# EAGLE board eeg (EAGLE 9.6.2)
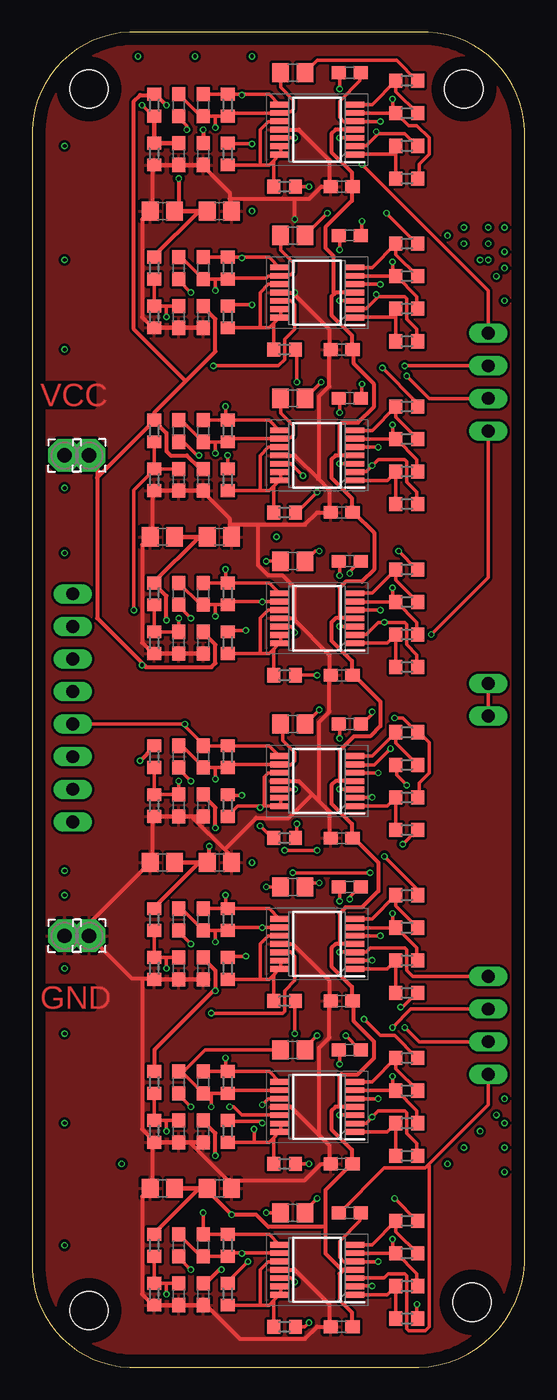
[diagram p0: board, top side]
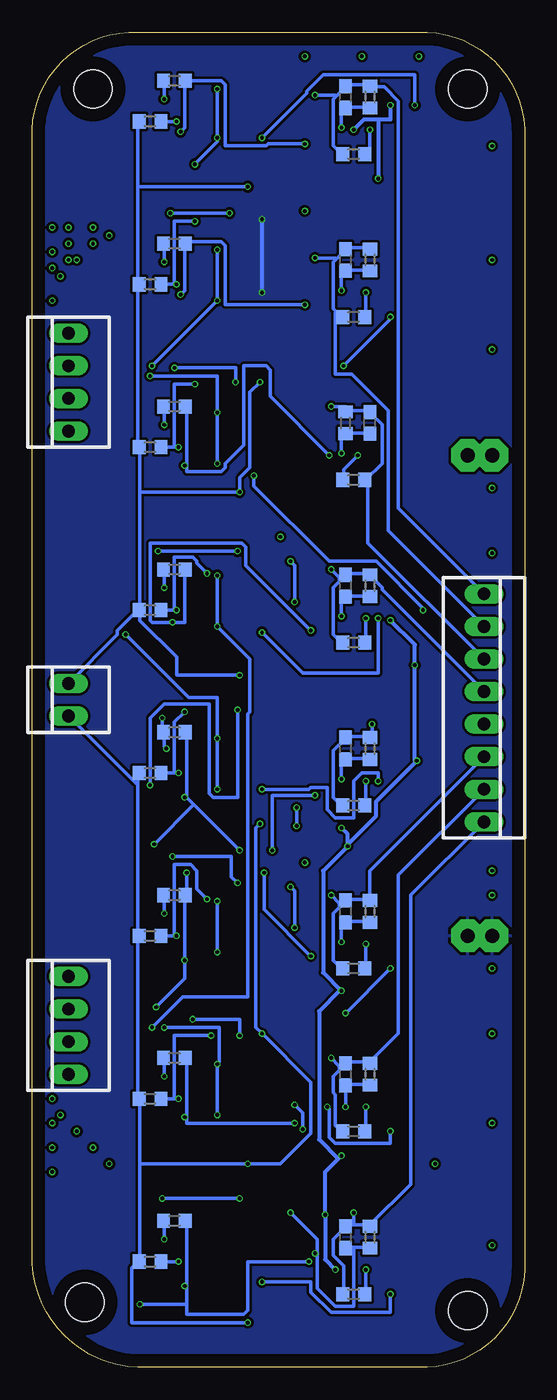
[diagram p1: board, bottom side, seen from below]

Size 38.4 x 104.13 mm. Coordinates in mm from the lower left corner, seen from the top.
Outline: 0,95.88 0,8.26 arc90 7.62,0 30.15,0 arc90 38.4,8.89 38.4,96.51 arc90 30.15,104.13 7.62,104.13 arc90 0,95.88
Copper layers (1*16): Top 0.035mm / dielectric 1.5mm / Bottom 0.035mm
Design rules "default *": minimum track width 10mil, minimum drill 0.3mm, track to track 6mil, track to pad 6mil, pad to pad 6mil, via to via 6mil, smd to smd 6mil, copper to edge 40mil, drill to drill 6mil, minimum pad ring 10mil, minimum via ring 2mil, stop-mask expansion 4mil, vias tented up to drill 0mil, thermal gap 10mil
Net classes: 0 default: width 0.254 mm, drill 0.3 mm, clearance 0.205 mm; 1 VCC: width 0.305 mm, drill 0.3 mm, clearance 0.205 mm; 2 GND: width 0.305 mm, drill 0.3 mm, clearance 0.205 mm
Holes 3 mm at 4.45,4.45 34.29,5.08 33.65,99.7 4.45,99.7

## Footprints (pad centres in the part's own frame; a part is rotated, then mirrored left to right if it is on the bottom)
22-23-2081 = drill 1 long: 1 -8.89,0; 2 -6.35,0; 3 -3.81,0; 4 -1.27,0; 5 1.27,0; 6 3.81,0; 7 6.35,0; 8 8.89,0
R0603 = smd 1 x 1.1: 1 -0.85,0; 2 0.85,0
C0603 = smd 1.1 x 1: 1 -0.85,0; 2 0.85,0
C0805 = smd 1.3 x 1.5: 1 -0.95,0; 2 0.95,0
22-23-2041 = drill 1 long: 1 -3.81,0; 2 -1.27,0; 3 1.27,0; 4 3.81,0
SOP65P640X120-14N = smd 1.475 x 0.45: 1 -2.938,1.95; 2 -2.938,1.3; 3 -2.938,0.65; 4 -2.938,0; 5 -2.938,-0.65; 6 -2.938,-1.3; 7 -2.938,-1.95; 8 2.938,-1.95; 9 2.938,-1.3; 10 2.938,-0.65; 11 2.938,0; 12 2.938,0.65; 13 2.938,1.3; 14 2.938,1.95
2,54/1,1 = drill 1.118 pad 2.54 octagon: 1 0,0
22-23-2021 = drill 1 long: 1 -1.27,0; 2 1.27,0

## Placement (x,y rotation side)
ANALOGOUT  22-23-2081  [22-23-2081]  3.18,51.44 270 bottom
BANDPASS  [R0603]  13.34,94.61 0 bottom
BANDPASS1  [R0603]  13.34,81.92 0 bottom
BANDPASS2  [R0603]  13.34,69.22 180 bottom
BANDPASS3  [R0603]  13.34,56.52 0 bottom
BANDPASS4  [R0603]  13.34,43.82 0 bottom
BANDPASS5  [R0603]  13.34,31.12 0 bottom
BANDPASS6  [R0603]  13.34,18.41 0 bottom
BANDPASS7  [R0603]  13.34,5.71 0 bottom
C1  [C0603]  24.77,100.97 0 top
C2  [C0603]  24.13,92.08 180 top
C3  [C0805]  20.32,100.97 0 top
C4  [C0603]  13.34,98.42 90 top
C5  [C0603]  13.34,94.61 270 top
C6  [C0603]  11.43,98.42 270 top
C7  [C0603]  11.43,94.61 270 top
C8  [C0805]  20.32,88.27 0 top
C9  [C0603]  24.77,88.27 0 top
C10  [C0603]  24.13,79.38 180 top
C11  [C0603]  13.34,81.92 270 top
C12  [C0603]  11.43,85.73 270 top
C13  [C0603]  13.34,85.73 90 top
C14  [C0603]  11.43,81.92 270 top
C15  [C0805]  20.32,75.56 0 top
C16  [C0603]  24.77,75.56 0 top
C17  [C0603]  24.13,66.67 180 top
C18  [C0603]  13.34,69.22 270 top
C19  [C0603]  11.43,73.03 270 top
C20  [C0603]  13.34,73.03 90 top
C21  [C0603]  11.43,69.22 270 top
C22  [C0805]  20.32,62.86 0 top
C23  [C0603]  24.77,62.86 0 top
C24  [C0603]  24.13,53.98 180 top
C25  [C0603]  13.34,56.52 270 top
C26  [C0603]  11.43,60.33 270 top
C27  [C0603]  13.34,60.33 90 top
C28  [C0603]  11.43,56.52 270 top
C29  [C0805]  20.32,50.16 0 top
C30  [C0603]  24.77,50.16 0 top
C31  [C0603]  24.13,41.27 180 top
C32  [C0603]  13.34,43.82 270 top
C33  [C0603]  11.43,47.62 270 top
C34  [C0603]  13.34,47.62 90 top
C35  [C0603]  11.43,43.82 270 top
C36  [C0805]  20.32,37.47 0 top
C37  [C0603]  24.77,37.47 0 top
C38  [C0603]  24.13,28.58 180 top
C39  [C0603]  13.34,31.12 270 top
C40  [C0603]  11.43,34.93 270 top
C41  [C0603]  13.34,34.93 90 top
C42  [C0603]  11.43,31.12 270 top
C43  [C0805]  20.32,24.77 0 top
C44  [C0603]  24.77,24.77 0 top
C45  [C0603]  24.13,15.87 180 top
C46  [C0603]  13.34,18.41 270 top
C47  [C0603]  11.43,22.23 270 top
C48  [C0603]  13.34,22.23 90 top
C49  [C0603]  11.43,18.41 270 top
C50  [C0805]  20.32,12.06 0 top
C51  [C0603]  24.77,12.06 0 top
C52  [C0603]  13.34,5.71 270 top
C53  [C0603]  24.13,3.18 180 top
C54  [C0603]  11.43,9.53 270 top
C55  [C0603]  13.34,9.53 90 top
C56  [C0603]  11.43,5.71 270 top
C59  [C0805]  10.16,90.17 180 top
C60  [C0805]  14.61,90.17 180 top
C61  [C0805]  10.16,64.77 180 top
C62  [C0805]  14.61,64.77 180 top
C63  [C0805]  10.16,39.37 180 top
C64  [C0805]  14.61,39.37 180 top
C65  [C0805]  10.16,13.97 180 top
C66  [C0805]  14.61,13.97 180 top
E$1  [22-23-2041]  35.56,76.84 90 bottom
E$2  [22-23-2041]  35.56,26.67 90 bottom
FILTERC  [C0603]  13.97,99.06 90 bottom
FILTERC1  [C0603]  13.97,86.36 90 bottom
FILTERC2  [C0603]  12.07,73.66 90 bottom
FILTERC3  [C0603]  13.97,60.96 90 bottom
FILTERC4  [C0603]  13.97,48.26 90 bottom
FILTERC5  [C0603]  13.97,35.56 90 bottom
FILTERC6  [C0603]  13.97,22.86 90 bottom
FILTERC7  [C0603]  13.97,10.16 90 bottom
FILTERR  [R0603]  12.07,99.06 270 bottom
FILTERR1  [R0603]  12.07,86.36 270 bottom
FILTERR2  [R0603]  13.97,73.66 270 bottom
FILTERR3  [R0603]  12.07,60.96 270 bottom
FILTERR4  [R0603]  12.07,48.26 270 bottom
FILTERR5  [R0603]  12.07,35.56 270 bottom
FILTERR6  [R0603]  12.07,22.86 270 bottom
FILTERR7  [R0603]  12.07,10.16 270 bottom
GAIN  [R0603]  27.3,100.33 180 bottom
GAIN1  [R0603]  27.3,87.63 180 bottom
GAIN2  [R0603]  27.3,74.93 180 bottom
GAIN3  [R0603]  27.3,62.23 180 bottom
GAIN4  [R0603]  27.3,49.53 180 bottom
GAIN5  [R0603]  27.3,36.83 180 bottom
GAIN6  [R0603]  27.3,24.13 180 bottom
GAIN7  [R0603]  27.3,11.43 180 bottom
IC1  ADTL084ARUZ  [SOP65P640X120-14N]  22.23,96.52 180 top
IC2  ADTL084ARUZ  [SOP65P640X120-14N]  22.23,83.82 180 top
IC3  ADTL084ARUZ  [SOP65P640X120-14N]  22.23,71.12 180 top
IC4  ADTL084ARUZ  [SOP65P640X120-14N]  22.23,58.42 180 top
IC5  ADTL084ARUZ  [SOP65P640X120-14N]  22.23,45.72 180 top
IC6  ADTL084ARUZ  [SOP65P640X120-14N]  22.23,33.02 180 top
IC7  ADTL084ARUZ  [SOP65P640X120-14N]  22.23,20.32 180 top
IC8  ADTL084ARUZ  [SOP65P640X120-14N]  22.23,7.62 180 top
PAD1  [2,54/1,1]  2.54,33.66 90 top
PAD2  [2,54/1,1]  4.45,33.66 90 top
PAD3  [2,54/1,1]  2.54,71.12 90 top
PAD4  [2,54/1,1]  4.45,71.12 90 top
R1  [R0603]  29.21,100.33 180 top
R2  [R0603]  29.21,97.79 0 top
R3  [R0603]  29.21,87.63 180 top
R4  [R0603]  29.21,85.09 0 top
R5  [R0603]  29.21,95.25 180 top
R6  [R0603]  29.21,92.71 180 top
R7  [R0603]  19.68,92.08 180 top
R8  [R0603]  15.24,98.42 270 top
R9  [R0603]  15.24,94.61 270 top
R10  [R0603]  9.53,98.42 270 top
R11  [R0603]  9.53,94.61 270 top
R12  [R0603]  29.21,82.55 180 top
R13  [R0603]  29.21,80.01 180 top
R14  [R0603]  15.24,81.92 270 top
R15  [R0603]  15.24,85.73 270 top
R16  [R0603]  9.53,85.73 270 top
R17  [R0603]  9.53,81.92 270 top
R18  [R0603]  19.68,79.38 180 top
R19  [R0603]  29.21,74.93 180 top
R20  [R0603]  29.21,72.39 0 top
R21  [R0603]  29.21,69.85 180 top
R22  [R0603]  29.21,67.31 180 top
R23  [R0603]  15.24,69.22 270 top
R24  [R0603]  15.24,73.03 270 top
R25  [R0603]  9.53,73.03 270 top
R26  [R0603]  9.53,69.22 270 top
R27  [R0603]  19.68,66.67 180 top
R28  [R0603]  29.21,62.23 180 top
R29  [R0603]  29.21,59.69 0 top
R30  [R0603]  29.21,57.15 180 top
R31  [R0603]  29.21,54.61 180 top
R32  [R0603]  15.24,56.52 270 top
R33  [R0603]  15.24,60.33 270 top
R34  [R0603]  9.53,60.33 270 top
R35  [R0603]  9.53,56.52 270 top
R36  [R0603]  19.68,53.98 180 top
R37  [R0603]  29.21,46.99 0 top
R38  [R0603]  29.21,49.53 180 top
R39  [R0603]  29.21,44.45 180 top
R40  [R0603]  29.21,41.91 180 top
R41  [R0603]  15.24,43.82 270 top
R42  [R0603]  15.24,47.62 270 top
R43  [R0603]  9.53,47.62 270 top
R44  [R0603]  9.53,43.82 270 top
R45  [R0603]  19.68,41.27 180 top
R46  [R0603]  29.21,36.83 180 top
R47  [R0603]  29.21,34.29 0 top
R48  [R0603]  29.21,31.75 180 top
R49  [R0603]  29.21,29.21 180 top
R50  [R0603]  15.24,31.12 270 top
R51  [R0603]  15.24,34.93 270 top
R52  [R0603]  9.53,34.93 270 top
R53  [R0603]  9.53,31.12 270 top
R54  [R0603]  19.68,28.58 180 top
R55  [R0603]  29.21,24.13 180 top
R56  [R0603]  29.21,21.59 0 top
R57  [R0603]  29.21,19.05 180 top
R58  [R0603]  29.21,16.51 180 top
R59  [R0603]  15.24,18.41 270 top
R60  [R0603]  15.24,22.23 270 top
R61  [R0603]  9.53,22.23 270 top
R62  [R0603]  9.53,18.41 270 top
R63  [R0603]  19.68,15.87 180 top
R64  [R0603]  29.21,11.43 180 top
R65  [R0603]  29.21,8.89 0 top
R66  [R0603]  29.21,6.35 180 top
R67  [R0603]  29.21,3.81 180 top
R68  [R0603]  15.24,5.71 270 top
R69  [R0603]  15.24,9.53 270 top
R70  [R0603]  9.53,9.53 270 top
R71  [R0603]  9.53,5.71 270 top
R72  [R0603]  19.68,3.18 180 top
R73  [R0603]  29.21,84.45 180 bottom
R74  [R0603]  29.21,97.16 180 bottom
R75  [R0603]  29.21,71.75 180 bottom
R76  [R0603]  29.21,59.06 180 bottom
R77  [R0603]  29.21,8.26 180 bottom
R78  [R0603]  29.21,20.95 180 bottom
R79  [R0603]  29.21,33.66 180 bottom
R80  [R0603]  29.21,46.36 180 bottom
REFERENCE  22-23-2021  [22-23-2021]  35.56,52.07 90 bottom

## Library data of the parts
ANALOGOUT = con-molex; MF: MOLEX; MPN: 22-23-2081; OC_FARNELL: 1756826; OC_NEWARK: 01C7592
BANDPASS BANDPASS1-BANDPASS7 FILTERR FILTERR1-FILTERR7 GAIN GAIN1-GAIN7 R1-R80 = rcl; SPICEPREFIX: R
C1-C56 C59-C66 FILTERC FILTERC1-FILTERC7 = rcl; SPICEPREFIX: C
E$1 E$2 = con-molex
IC1-IC8 = ADTL084ARUZ; ARROW_PART_NUMBER: ADTL084ARUZ; ARROW_PRICE-STOCK: https://www.arrow.com/en/products/adtl084aruz/analog-devices; DESCRIPTION: ADTL084ARUZ, Quad Operational Amplifier 5MHz, 14-Pin TSSOP; HEIGHT: 1.2mm; MANUFACTURER_NAME: Analog Devices; MANUFACTURER_PART_NUMBER: ADTL084ARUZ; MOUSER_PART_NUMBER: 584-ADTL084ARUZ; MOUSER_PRICE-STOCK: https://www.mouser.co.uk/ProductDetail/Analog-Devices/ADTL084ARUZ?qs=WIvQP4zGanh2v1vzKZRzoA%3D%3D
PAD1-PAD4 = wirepad
REFERENCE = con-molex; MF: MOLEX; MPN: 22-23-2021; OC_FARNELL: 1462926; OC_NEWARK: 25C3832

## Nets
ADC1: ANALOGOUT.1 BANDPASS.1 C4.2 FILTERC.2 FILTERR.1 IC1.8 R8.1
ADC2: ANALOGOUT.2 BANDPASS1.1 C13.2 FILTERC1.2 FILTERR1.1 IC2.8 R15.1
ADC3: ANALOGOUT.3 BANDPASS2.1 C20.2 FILTERC2.2 FILTERR2.1 IC3.8 R24.1
ADC4: ANALOGOUT.4 BANDPASS3.1 C27.2 FILTERC3.2 FILTERR3.1 IC4.8 R33.1
ADC5: ANALOGOUT.5 BANDPASS4.1 C34.2 FILTERC4.2 FILTERR4.1 IC5.8 R42.1
ADC6: ANALOGOUT.6 BANDPASS5.1 C41.2 FILTERC5.2 FILTERR5.1 IC6.8 R51.1
ADC7: ANALOGOUT.7 BANDPASS6.1 C48.2 FILTERC6.2 FILTERR6.1 IC7.8 R60.1
ADC8: ANALOGOUT.8 BANDPASS7.1 C55.2 FILTERC7.2 FILTERR7.1 IC8.8 R69.1
B$1: C3.1 C4.1 C6.1 FILTERC.1 FILTERR.2 IC1.9 R8.2
B$2: C8.1 C12.1 C13.1 FILTERC1.1 FILTERR1.2 IC2.9 R15.2
B$3: C15.1 C19.1 C20.1 FILTERC2.1 FILTERR2.2 IC3.9 R24.2
B$4: C22.1 C26.1 C27.1 FILTERC3.1 FILTERR3.2 IC4.9 R33.2
B$5: C29.1 C33.1 C34.1 FILTERC4.1 FILTERR4.2 IC5.9 R42.2
B$6: C36.1 C40.1 C41.1 FILTERC5.1 FILTERR5.2 IC6.9 R51.2
B$7: C43.1 C47.1 C48.1 FILTERC6.1 FILTERR6.2 IC7.9 R60.2
B$8: C50.1 C54.1 C55.1 FILTERC7.1 FILTERR7.2 IC8.9 R69.2
GND [GND]: C2.2 C5.2 C7.2 C10.2 C11.2 C14.2 C17.2 C18.2 C21.2 C24.2 C25.2 C28.2 C31.2 C32.2 C35.2 C38.2 C39.2 C42.2 C45.2 C46.2 C49.2 C52.2 C53.2 C56.2 C59.2 C60.1 C61.2 C62.1 C63.2 C64.1 C65.2 C66.1 IC1.11 IC2.11 IC3.11 IC4.11 IC5.11 IC6.11 IC7.11 IC8.11 PAD1.1 PAD2.1 R11.2 R17.2 R26.2 R35.2 R44.2 R53.2 R62.2 R71.2
IN1+: C1.1 E$1.4 IC1.3
IN2+: C9.1 E$1.3 IC2.3
IN2-: C9.2 IC2.5 R73.1
IN3+: C16.1 E$1.2 IC3.3
IN4+: C23.1 E$2.2 IC4.3
IN5+: C30.1 E$1.1 IC5.3
IN6+: C37.1 E$2.4 IC6.3
IN7+: C44.1 E$2.3 IC7.3
IN8+: C51.1 E$2.1 IC8.3
N$1: IC1.7 R1.2 R2.2
N$2: C3.2 R1.1
N$3: GAIN.2 IC1.6 R2.1 R6.1
N$4: IC1.1 R5.2 R6.2
N$5: IC2.7 R3.2 R4.2
N$6: IC1.10 IC1.13 IC1.14 R7.2 R9.2
N$7: GAIN.1 IC1.2 R5.1 R9.1
N$8: GAIN1.2 IC2.6 R4.1 R12.1
N$9: IC2.1 R12.2 R13.2
N$10: IC2.10 IC2.13 IC2.14 R14.2 R18.2
N$11: BANDPASS.2 C6.2
N$12: C7.1 IC1.12 R10.2 R11.1
N$13: GAIN1.1 IC2.2 R13.1 R14.1
N$14: C8.2 R3.1
N$15: BANDPASS1.2 C12.2
N$16: C14.1 IC2.12 R16.2 R17.1
N$17: IC3.7 R19.2 R20.2
N$18: GAIN2.2 IC3.6 R20.1 R21.1
N$19: IC3.1 R21.2 R22.2
N$20: IC3.10 IC3.13 IC3.14 R23.2 R27.2
N$21: GAIN2.1 IC3.2 R22.1 R23.1
N$22: C15.2 R19.1
N$23: BANDPASS2.2 C19.2
N$24: C21.1 IC3.12 R25.2 R26.1
N$25: IC4.7 R28.2 R29.2
N$26: GAIN3.2 IC4.6 R29.1 R30.1
N$27: IC4.1 R30.2 R31.2
N$28: IC4.10 IC4.13 IC4.14 R32.2 R36.2
N$29: GAIN3.1 IC4.2 R31.1 R32.1
N$30: C22.2 R28.1
N$31: BANDPASS3.2 C26.2
N$32: C28.1 IC4.12 R34.2 R35.1
N$33: IC5.7 R37.2 R38.2
N$34: GAIN4.2 IC5.6 R38.1 R39.1
N$35: IC5.1 R39.2 R40.2
N$36: IC5.10 IC5.13 IC5.14 R41.2 R45.2
N$37: GAIN4.1 IC5.2 R40.1 R41.1
N$38: C29.2 R37.1
N$39: BANDPASS4.2 C33.2
N$40: C35.1 IC5.12 R43.2 R44.1
N$41: IC6.7 R46.2 R47.2
N$42: GAIN5.2 IC6.6 R47.1 R48.1
N$43: IC6.1 R48.2 R49.2
N$44: IC6.10 IC6.13 IC6.14 R50.2 R54.2
N$45: GAIN5.1 IC6.2 R49.1 R50.1
N$46: C36.2 R46.1
N$47: BANDPASS5.2 C40.2
N$48: C42.1 IC6.12 R52.2 R53.1
N$49: IC7.7 R55.2 R56.2
N$50: GAIN6.2 IC7.6 R56.1 R57.1
N$51: IC7.1 R57.2 R58.2
N$52: IC7.10 IC7.13 IC7.14 R59.2 R63.2
N$53: GAIN6.1 IC7.2 R58.1 R59.1
N$54: C43.2 R55.1
N$55: BANDPASS6.2 C47.2
N$56: C49.1 IC7.12 R61.2 R62.1
N$57: IC8.7 R64.2 R65.2
N$58: GAIN7.2 IC8.6 R65.1 R66.1
N$59: IC8.1 R66.2 R67.2
N$60: IC8.10 IC8.13 IC8.14 R68.2 R72.2
N$61: GAIN7.1 IC8.2 R67.1 R68.1
N$62: C50.2 R64.1
N$63: BANDPASS7.2 C54.2
N$64: C56.1 IC8.12 R70.2 R71.1
N$65: C1.2 IC1.5 R74.1
N$67: C51.2 IC8.5 R77.1
N$68: C44.2 IC7.5 R78.1
N$69: C37.2 IC6.5 R79.1
N$70: C30.2 IC5.5 R80.1
N$71: C23.2 IC4.5 R76.1
N$72: C16.2 IC3.5 R75.1
REF: R7.1 R18.1 R27.1 R36.1 R45.1 R54.1 R63.1 R72.1 R73.2 R74.2 R75.2 R76.2 R77.2 R78.2 R79.2 R80.2 REFERENCE.1 REFERENCE.2
VCC [VCC]: C2.1 C5.1 C10.1 C11.1 C17.1 C18.1 C24.1 C25.1 C31.1 C32.1 C38.1 C39.1 C45.1 C46.1 C52.1 C53.1 C59.1 C60.2 C61.1 C62.2 C63.1 C64.2 C65.1 C66.2 IC1.4 IC2.4 IC3.4 IC4.4 IC5.4 IC6.4 IC7.4 IC8.4 PAD3.1 PAD4.1 R10.1 R16.1 R25.1 R34.1 R43.1 R52.1 R61.1 R70.1

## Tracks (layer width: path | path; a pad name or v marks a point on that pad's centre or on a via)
ADC1  (via drill 0.3)
  Top 0.254: IC1.8 18.48,99.28 16.35,99.28 | 16.35,99.28 R8.1 C4.2 | v16.35,99.22 16.35,99.28
  Bottom 0.254: 14.68,99.14 13.97,99.85 FILTERC.2 13.97,100.01 12.07,100.01 FILTERR.1 12.07,99.85 10.95,99.85 9.84,98.74 9.84,66.99 ANALOGOUT.1 | 14.68,99.14 14.92,98.9 14.92,95.25 14.29,94.61 BANDPASS.1 | v16.35,99.22 14.76,99.22 14.68,99.14
ADC2  (via drill 0.3)
  Top 0.254: IC2.8 18.48,86.58 16.35,86.58 | 16.35,86.58 R15.1 C13.2 | v16.35,86.52 16.35,86.58
  Bottom 0.254: FILTERR1.1 12.07,87.31 13.97,87.31 FILTERC1.2 13.97,87.15 14.68,86.44 | 14.68,82.31 14.92,82.55 14.92,86.2 14.68,86.44 | 14.68,82.31 14.29,81.92 BANDPASS1.1 | ANALOGOUT.2 10.64,65.25 10.64,74.61 13.49,77.47 14.76,77.47 14.76,82.23 14.68,82.31 | v16.35,86.52 14.76,86.52 14.68,86.44
ADC3  (via drill 0.3)
  Top 0.254: R24.1 C20.2 | R24.1 18.48,73.88 IC3.8 | v15.08,74.93 15.08,73.98 R24.1
  Bottom 0.254: 13.97,74.61 12.07,74.61 FILTERC2.2 12.07,74.45 11.11,73.5 11.11,70.48 12.38,69.22 BANDPASS2.1 12.22,69.22 12.22,64.29 ANALOGOUT.3 | v15.08,74.93 13.97,74.93 13.97,74.61 | 13.97,74.61 FILTERR2.1
ADC4  (via drill 0.3)
  Top 0.254: IC4.8 18.48,61.17 R33.1 | R33.1 C27.2 | v15.08,62.23 15.08,61.28 R33.1
  Bottom 0.254: FILTERC3.2 13.97,61.91 12.07,61.91 FILTERR3.1 12.07,61.75 11.11,60.8 11.11,60.64 ANALOGOUT.4 | BANDPASS3.1 14.29,56.52 14.92,57.15 14.92,60.8 13.97,61.75 FILTERC3.2 | v15.08,62.23 14.45,61.59 14.45,61.44 FILTERC3.2
ADC5  (via drill 0.3)
  Top 0.254: IC5.8 18.48,48.48 R42.1 C34.2 13.34,48.58 11.83,50.09 | ANALOGOUT.5 11.75,50.16 11.83,50.09 | v11.91,50.16 11.83,50.09
  Bottom 0.254: 12.07,49.21 13.97,49.21 FILTERC4.2 13.97,49.05 14.92,48.1 14.92,44.45 14.29,43.82 BANDPASS4.1 | 12.07,49.21 11.91,49.37 v11.91,50.16 | 12.07,49.21 FILTERR4.1
ADC6  (via drill 0.3)
  Top 0.254: IC6.8 18.48,35.77 R51.1 | R51.1 C41.2 | v15.08,36.83 15.08,35.88 R51.1
  Bottom 0.254: 12.07,36.51 13.97,36.51 FILTERC5.2 | BANDPASS5.1 14.29,31.12 14.92,31.75 14.92,35.4 13.97,36.35 FILTERC5.2 | ANALOGOUT.6 12.07,38.73 12.07,36.51 | 12.07,36.51 FILTERR5.1 | v15.08,36.83 14.45,36.2 14.45,36.04 FILTERC5.2
ADC7  (via drill 0.3)
  Top 0.254: IC7.8 18.48,23.08 R60.1 | R60.1 C48.2 | v15.08,24.13 15.08,23.18 R60.1
  Bottom 0.254: 12.07,23.81 13.97,23.81 FILTERC6.2 | BANDPASS6.1 14.29,18.41 14.76,18.89 14.76,21.27 14.92,21.43 14.92,22.7 13.97,23.65 FILTERC6.2 | ANALOGOUT.7 9.84,38.42 9.84,26.03 12.07,23.81 | 12.07,23.81 FILTERR6.1 | v15.08,24.13 14.45,23.49 14.45,23.34 FILTERC6.2
ADC8  (via drill 0.3)
  Top 0.254: IC8.8 18.48,10.38 R69.1 C55.2 v13.34,12.06
  Bottom 0.254: 13.34,11.11 13.97,11.11 FILTERC7.2 13.97,10.95 14.92,10 14.92,8.73 14.13,7.94 14.13,5.71 BANDPASS7.1 | 13.34,11.11 12.07,11.11 | ANALOGOUT.8 8.89,36.83 8.89,14.29 12.07,11.11 | 12.07,11.11 FILTERR7.1 | 13.34,11.11 v13.34,12.06
B$1  (via drill 0.3)
  Top 0.254: C6.1 13.13,97.58 C4.1 14.29,97.58 | 14.29,97.58 R8.2 15.48,97.82 IC1.9 19.38,97.91 20.16,97.91 20.36,98.11 20.36,98.83 19.37,99.82 C3.1 | 14.29,97.58 v14.29,96.68
  Bottom 0.254: FILTERR.2 12.07,98.27 13.97,98.27 FILTERC.1 13.97,98.11 14.29,97.79 v14.29,96.68
B$2  (via drill 0.3)
  Top 0.254: C8.1 19.37,87.12 20.36,86.13 20.36,85.41 20.16,85.21 19.38,85.21 IC2.9 19.21,85.09 18.41,85.09 18.26,84.93 15.24,84.93 R15.2 14.29,84.88 | 14.29,84.88 C13.1 11.63,86.58 C12.1 | 14.29,84.88 v14.29,83.98
  Bottom 0.254: FILTERR1.2 12.07,85.57 13.97,85.57 FILTERC1.1 13.97,85.41 14.29,85.09 v14.29,83.98
B$3  (via drill 0.3)
  Top 0.254: C15.1 19.37,74.42 20.36,73.43 20.36,72.71 20.16,72.51 19.38,72.51 IC3.9 15.48,72.42 R24.2 14.29,72.17 | C19.1 11.63,73.88 C20.1 14.29,72.17 | 14.29,72.17 v14.29,71.28
  Bottom 0.254: FILTERC2.1 12.07,72.87 13.97,72.87 FILTERR2.2 13.97,72.71 14.29,72.39 v14.29,71.28
B$4  (via drill 0.3)
  Top 0.254: C26.1 13.13,59.48 C27.1 14.29,59.48 | 14.29,59.48 R33.2 15.48,59.72 17.94,59.72 | IC4.9 17.94,59.72 | v18.26,62.86 C22.1 | v17.94,59.69 17.94,59.72 | 14.29,59.48 v14.29,58.58
  Bottom 0.254: FILTERR3.2 12.07,60.17 13.97,60.17 FILTERC3.1 13.97,60.01 14.29,59.69 v14.29,58.58 | v18.26,62.86 17.94,62.55 v17.94,59.69
B$5  (via drill 0.3)
  Top 0.254: 14.29,46.77 C34.1 13.34,46.83 11.75,48.42 11.43,48.42 C33.1 | 14.29,46.77 R42.2 15.48,47.02 IC5.9 19.37,46.99 20.16,46.99 20.48,47.31 20.48,47.94 19.53,48.9 19.53,50.16 C29.1 | 14.29,46.77 v14.29,45.88
  Bottom 0.254: FILTERR4.2 12.07,47.47 13.97,47.47 FILTERC4.1 13.97,47.31 14.29,46.99 v14.29,45.88
B$6  (via drill 0.3)
  Top 0.254: 14.29,34.08 C41.1 11.63,35.77 C40.1 | 14.29,34.08 R51.2 15.48,34.32 17.94,34.32 | 17.94,34.32 IC6.9 | v18.26,37.47 C36.1 | v17.94,34.29 17.94,34.32 | 14.29,34.08 v14.29,33.18
  Bottom 0.254: FILTERR5.2 12.07,34.77 13.97,34.77 FILTERC5.1 13.97,34.61 14.29,34.29 v14.29,33.18 | v18.26,37.47 17.94,37.15 v17.94,34.29
B$7  (via drill 0.3)
  Top 0.254: 13.97,21.38 C48.1 11.63,23.08 C47.1 11.75,23.02 13.49,24.77 C43.1 | 13.97,21.38 R60.2 15.48,21.62 IC7.9 | 13.97,21.38 v13.97,20.32
  Bottom 0.254: FILTERR6.2 12.07,22.07 13.97,22.07 FILTERC6.1 v13.97,20.32
B$8  (via drill 0.3)
  Top 0.254: C54.1 13.13,8.68 C55.1 R69.2 15.48,8.92 16.35,8.92 | 16.35,8.92 IC8.9 | v18.26,12.06 C50.1 | v16.35,8.89 16.35,8.92
  Bottom 0.254: 13.34,9.37 13.97,9.37 FILTERC7.1 | 13.34,9.37 12.07,9.37 FILTERR7.2 | v18.26,12.06 16.19,10 16.19,8.89 | 16.19,8.89 16.19,6.19 14.76,4.76 13.34,4.76 13.34,9.37 | 16.19,8.89 v16.35,8.89
GND  (via drill 0.3)
  Top 0.305: 23.18,92.08 23.18,94.14 20.8,96.52 IC1.11 | R11.2 9.37,93.82 9.37,90.17 C59.2 8.57,89.53 8.57,81.92 9.37,81.12 R17.2 | 15.4,91.12 15.4,91.6 13.34,93.66 C5.2 | 15.4,91.12 15.4,90.17 C60.1 | 23.18,92.08 22.54,92.08 21.59,91.12 20.48,91.12 | 15.4,91.12 20.48,91.12 | 23.18,92.08 C2.2 | 23.18,79.38 23.18,80.96 20.4,83.74 | 20.4,83.74 20.32,83.82 IC2.11 | 23.18,66.67 23.18,68.42 22.3,69.29 | 22.3,69.29 20.48,71.12 IC3.11 | R26.2 9.37,68.42 9.37,64.77 C61.2 8.57,64.14 8.57,56.52 9.37,55.72 R35.2 | 15.4,65.72 15.4,66.2 13.34,68.26 C18.2 | 15.4,65.72 15.4,64.77 C62.1 | 23.18,66.67 22.23,66.67 21.27,65.72 17.62,65.72 | 15.4,65.72 17.62,65.72 | 23.18,66.67 C17.2 | 23.18,79.38 23.18,76.52 22.38,75.72 22.38,69.37 22.3,69.29 | 23.18,79.38 C10.2 | v20.48,89.53 20.48,91.12 | v20.48,83.82 20.4,83.74 | 23.18,28.58 23.18,30.16 20.32,33.02 IC6.11 | 23.18,15.87 23.18,17.3 22.3,18.18 | 22.3,18.18 20.16,20.32 IC7.11 | 23.18,3.18 23.18,4.92 20.48,7.62 IC8.11 | 12.38,17.56 12.38,17.46 15.4,14.45 15.4,13.97 C66.1 15.4,14.6 21.27,14.6 22.54,15.87 23.18,15.87 | R71.2 9.37,4.92 8.57,5.71 8.57,13.33 C65.2 9.37,13.97 9.37,17.62 R62.2 9.37,17.78 8.57,18.57 8.57,30.32 | 23.18,3.18 22.23,3.18 21.27,2.22 16.19,2.22 13.49,4.92 C52.2 | 23.18,3.18 C53.2 | 23.18,15.87 C45.2 | 23.18,28.58 23.18,25.72 22.38,24.92 22.38,18.26 22.3,18.18 | 23.18,28.58 C38.2 | 8.57,30.32 7.78,30.32 PAD2.1 | 8.57,30.32 9.37,30.32 R53.2 | PAD2.1 PAD1.1 | 23.18,53.98 23.18,55.56 20.4,58.34 | 20.4,58.34 20.32,58.42 IC4.11 | 21.83,44.69 20.8,45.72 IC5.11 | 21.83,44.69 22.3,44.21 | 22.3,44.21 23.18,43.34 23.18,41.27 C31.2 | R44.2 9.37,43.02 9.37,39.37 C63.2 4.6,34.77 4.6,33.66 PAD2.1
  Top 0.305: 15,40.4 12.54,42.86 12.54,42.97 | 15,40.4 15.4,40.01 15.4,39.37 C64.1 | 21.83,44.69 20,42.86 17.46,42.86 15,40.4 | 23.18,53.98 23.18,51.12 22.38,50.32 22.38,44.29 22.3,44.21 | 23.18,53.98 C24.2 | 17.62,65.72 17.62,62.55 18.41,61.75 19.53,61.75 20.48,60.8 20.48,58.42 20.4,58.34
  Top 0.356: R11.2 C7.2 C5.2 | R17.2 C14.2 C11.2 | C25.2 C28.2 R35.2 | R71.2 C56.2 C52.2 | R62.2 C49.2 12.38,17.56 C46.2 | R53.2 C42.2 C39.2 | R44.2 C35.2 12.54,42.97 C32.2 | R26.2 C21.2 C18.2
  Bottom 0.305: v20.48,83.82 v20.48,89.53
  pour Top: 7.62,104.14 31.75,104.14 arc-90 38.73,97.16 38.73,96.52 38.73,8.89 arc-90 29.84,0 22.23,0 7.62,0 arc-90 0,7.62 0,20.32 0,97.16 arc-90 6.99,104.14
  pour Bottom: 7.62,104.14 31.11,104.14 arc-90 38.73,96.52 38.73,8.89 38.73,8.26 arc-90 30.48,0 23.5,0 7.62,0 arc-90 0,7.62 0,20.95 0,97.79 arc-90 6.35,104.14
IN1+  (via drill 0.3)
  Top 0.254: v23.97,99.7 23.97,100.97 C1.1 | v23.97,95.89 25.08,95.89 IC1.3 | E$1.4 35.56,83.98 v25.72,93.82
  Bottom 0.254: v23.97,99.7 v23.97,95.89 23.97,95.57 v25.72,93.82
IN2+  (via drill 0.3)
  Top 0.254: v23.97,87.15 23.97,88.27 C9.1 | v23.97,83.19 25.08,83.19 IC2.3 | v29.05,78.11 E$1.3
  Bottom 0.254: v23.97,87.15 v23.97,83.19 v29.05,78.11
IN2-  (via drill 0.3)
  Top 0.254: v27.15,84.45 25.24,84.45 IC2.5 | v25.72,89.38 25.72,88.27 C9.2
  Bottom 0.254: 27.3,84.45 R73.1 | v25.72,89.38 27.3,89.38 27.3,84.45 | 27.3,84.45 v27.15,84.45
IN3+  (via drill 0.3)
  Top 0.254: v23.97,74.45 23.97,75.56 C16.1 | v23.97,70.48 25.08,70.48 IC3.3 | E$1.2 30.96,75.56 v29.21,77.31
  Bottom 0.254: v23.97,70.48 v23.97,74.45 23.97,77.31 v29.21,77.31
IN4+  (via drill 0.3)
  Top 0.254: v23.97,61.75 23.97,62.86 C23.1 | v23.97,57.79 25.08,57.79 IC4.3 | E$2.2 30.16,25.4 v29.05,26.51
  Bottom 0.254: v23.97,61.75 v23.97,57.79 21.43,55.25 21.43,51.12 21.59,50.96 21.59,28.89 26.67,28.89 v29.05,26.51
IN5+  (via drill 0.3)
  Top 0.254: v23.97,49.05 23.97,50.16 C30.1 | v23.97,45.09 25.08,45.09 IC5.3 | E$1.1 35.56,61.59 v31.11,57.15
  Bottom 0.254: v23.97,45.09 v23.97,49.05 23.97,52.23 26.19,52.23 v31.11,57.15
IN6+  (via drill 0.3)
  Top 0.254: v23.97,36.35 23.97,37.47 C37.1 | v23.97,32.39 25.08,32.39 IC6.3 25.24,32.39 26.04,32.39 26.35,32.7 29.05,32.7 29.21,32.54 29.21,30.96 29.69,30.48 E$2.4
  Bottom 0.254: v23.97,32.39 v23.97,36.35
IN7+  (via drill 0.3)
  Top 0.254: v23.97,23.65 23.97,24.77 C44.1 | v23.97,19.69 25.08,19.69 IC7.3 | E$2.3 29.53,27.94 v28.1,26.51
  Bottom 0.254: v23.97,19.69 v23.97,23.65 23.81,23.81 23.81,26.51 v28.1,26.51
IN8+
  Top 0.254: 30.88,15.8 35.56,20.48 E$2.1 | 30.88,15.8 30.64,15.56 27.46,15.56 23.97,12.06 C51.1 | IC8.3 25.24,6.98 27.46,6.98 27.78,7.3 29.05,7.3 29.21,7.14 29.21,3.02 29.37,2.86 30.64,2.86 30.96,3.18 30.96,15.72 30.88,15.8
N$1
  Top 0.254: IC1.7 26.5,98.47 R1.2 28.36,99.49 R2.2
N$2
  Top 0.254: R1.1 30,100.33 28.42,101.92 22.23,101.92 C3.2
N$3  (via drill 0.3)
  Top 0.254: R6.1 30.16,92.71 30.16,93.82 30.96,94.61 30.96,95.89 30,96.84 29.37,96.84 28.42,97.79 R2.1 | v28.1,98.9 28.1,97.95 28.26,97.79 R2.1 | R2.1 25.24,97.79 IC1.6
  Bottom 0.254: v28.1,98.9 28.1,100.33 GAIN.2
N$4
  Top 0.254: R6.2 28.36,94.61 | 28.36,94.61 R5.2 | IC1.1 25.21,94.61 28.36,94.61
N$5
  Top 0.254: R4.2 28.36,86.79 R3.2 26.5,85.77 IC2.7
N$6
  Top 0.254: R9.2 17.78,93.77 | 17.78,93.77 18.48,93.77 18.84,94.12 | R7.2 18.84,94.12 | 18.84,94.12 IC1.14 19.37,94.61 19.37,95.09 IC1.13 | 17.78,93.77 17.78,96.52 18.41,97.16 19.21,97.16 IC1.10
N$7  (via drill 0.3)
  Top 0.254: 26.91,96.12 26.04,95.25 25.24,95.25 IC1.2 | 26.91,96.12 26.99,96.2 29.05,96.2 30,95.25 R5.1 | v17.14,95.41 15.24,95.41 R9.1 | v26.83,96.36 26.83,96.2 26.91,96.12
  Bottom 0.254: v17.14,95.41 20,95.41 20.16,95.25 23.34,95.25 23.34,100.01 23.65,100.33 GAIN.1 26.51,100.33 26.51,96.68 v26.83,96.36
N$8  (via drill 0.3)
  Top 0.254: R12.1 30,82.55 30,83.5 28.42,85.09 R4.1 | v28.1,86.2 28.1,85.25 28.26,85.09 R4.1 | R4.1 25.24,85.09 IC2.6
  Bottom 0.254: v28.1,86.2 28.1,87.63 GAIN1.2
N$9
  Top 0.254: R13.2 28.36,81.92 | 28.36,81.92 R12.2 | IC2.1 25.21,81.92 28.36,81.92
N$10
  Top 0.254: R18.2 18.84,81.42 IC2.14 | R14.2 17.78,81.06 | 17.78,81.06 18.48,81.06 IC2.14 | IC2.13 19.37,82.39 19.37,81.92 IC2.14 | 17.78,81.06 17.78,83.82 18.41,84.45 19.21,84.45 IC2.10
N$11  (via drill 0.3)
  Top 0.254: v12.07,96.52 12.07,96.84 11.43,97.47 C6.2
  Bottom 0.254: v12.07,96.52 12.07,94.93 12.38,94.61 BANDPASS.2
N$12  (via drill 0.3)
  Top 0.254: v20.48,95.89 19.37,95.89 IC1.12 | v8.57,98.42 9.37,97.63 R10.2
  Top 0.356: R10.2 R11.1 C7.1
  Bottom 0.254: v20.48,95.89 16.99,99.38 16.99,99.54 15.72,100.81 8.57,100.81 v8.57,98.42
N$13  (via drill 0.3)
  Top 0.254: 26.91,83.42 26.04,82.55 25.24,82.55 IC2.2 | 26.91,83.42 26.99,83.5 29.05,83.5 29.21,83.34 29.21,81.76 30,80.96 30,80.01 R13.1 | v17.14,82.87 15.24,82.87 R14.1 | v26.83,83.66 26.83,83.5 26.91,83.42
  Bottom 0.254: v17.14,82.87 23.34,82.87 23.34,87.47 23.65,87.79 26.35,87.79 26.35,87.63 GAIN1.1 26.51,87.63 26.51,83.98 v26.83,83.66
N$14  (via drill 0.3)
  Top 0.254: v27.62,90.01 30,87.63 R3.1 | v23.02,90.01 C8.2
  Bottom 0.254: v23.02,90.01 v27.62,90.01
N$15  (via drill 0.3)
  Top 0.254: v12.38,83.82 11.43,84.77 C12.2
  Bottom 0.254: v12.38,83.82 12.38,81.92 BANDPASS1.2
N$16  (via drill 0.3)
  Top 0.254: R16.2 R17.1 10.48,82.77 | 10.48,82.77 C14.1 | v14.13,78.11 19.21,78.11 19.68,78.58 19.68,80.17 20.48,80.96 20.48,82.87 20.16,83.19 19.37,83.19 IC2.12 | 10.48,82.77 v10.48,81.92
  Bottom 0.254: v14.13,78.11 10.48,81.76 v10.48,81.92
N$17
  Top 0.254: IC3.7 26.5,73.07 R19.2 28.36,74.09 R20.2
N$18  (via drill 0.3)
  Top 0.254: R21.1 30,69.85 30,70.8 28.42,72.39 R20.1 | v28.1,73.5 28.1,72.55 28.26,72.39 R20.1 | R20.1 25.24,72.39 IC3.6
  Bottom 0.254: v28.1,73.5 28.1,74.93 GAIN2.2
N$19
  Top 0.254: IC3.1 27.68,69.17 28.15,69.64 | 28.15,69.64 R21.2 | R22.2 28.36,69.43 28.15,69.64
N$20
  Top 0.254: R27.2 18.84,68.72 IC3.14 | R23.2 17.78,68.36 | 17.78,68.36 18.48,68.36 IC3.14 | IC3.13 19.37,69.69 19.37,69.22 IC3.14 | 17.78,68.36 17.78,71.12 18.41,71.75 19.21,71.75 IC3.10
N$21  (via drill 0.3)
  Top 0.254: R22.1 30,67.31 30,68.26 29.21,69.06 29.21,70.64 29.05,70.8 26.99,70.8 v26.51,70.33 26.04,69.85 25.24,69.85 IC3.2 | v15.24,71.12 R23.1
  Bottom 0.254: v15.24,71.12 19.84,75.72 19.84,77.79 20.16,78.11 21.91,78.11 21.91,71.91 23.34,70.48 23.34,70.17 23.65,69.85 26.35,69.85 26.35,70.33 | 26.35,70.33 26.35,74.93 GAIN2.1 | 26.35,70.33 v26.51,70.33
N$22  (via drill 0.3)
  Top 0.254: v27.3,77.95 30,75.25 30,74.93 R19.1 | v22.54,76.84 C15.2
  Bottom 0.254: v27.3,77.95 22.54,77.95 v22.54,76.84
N$23  (via drill 0.3)
  Top 0.254: v13.02,71.12 12.86,71.12 11.91,72.07 11.43,72.07 C19.2
  Bottom 0.254: v13.02,71.12 14.13,70.01 14.13,69.22 BANDPASS2.2
N$24  (via drill 0.3)
  Top 0.254: R25.2 R26.1 | C21.1 R26.1 | v21.11,69.53 20.16,70.48 19.37,70.48 IC3.12 | v7.94,59.06 7.94,68.42 9.53,70.01 R26.1
  Bottom 0.254: v21.11,69.53 21.11,68.74 15.24,62.86 11.59,62.86 7.94,59.21 v7.94,59.06
N$25
  Top 0.254: IC4.7 26.5,60.37 R28.2 28.36,61.39 R29.2
N$26  (via drill 0.3)
  Top 0.254: R30.1 30,57.15 30,58.1 28.42,59.69 R29.1 | v28.1,60.8 28.1,59.85 28.26,59.69 R29.1 | R29.1 25.24,59.69 IC4.6
  Bottom 0.254: v28.1,60.8 28.1,62.23 GAIN3.2
N$27
  Top 0.254: IC4.1 27.68,56.47 R30.2 R31.2
N$28
  Top 0.254: R32.2 17.78,55.66 | 17.78,55.66 18.48,55.66 18.84,56.02 | R36.2 18.84,56.02 | 18.84,56.02 IC4.14 19.37,56.52 19.37,56.99 IC4.13 | 17.78,55.66 17.78,58.42 18.41,59.06 19.21,59.06 IC4.10
N$29  (via drill 0.3)
  Top 0.254: R31.1 30,54.61 30,55.56 29.21,56.36 29.21,57.94 29.05,58.1 v27.46,58.1 26.99,58.1 26.04,57.15 25.24,57.15 IC4.2 | v16.67,57.47 15.24,57.47 R32.1
  Bottom 0.254: v16.67,57.47 21.75,62.55 21.75,63.98 22.07,64.29 29.21,64.29 29.21,58.26 29.05,58.1 v27.46,58.1 26.51,58.1 26.51,62.23 GAIN3.1
N$30  (via drill 0.3)
  Top 0.254: v28.57,63.66 30,62.23 R28.1 | v22.38,63.66 22.07,63.66 C22.2
  Bottom 0.254: v22.38,63.66 v28.57,63.66
N$31  (via drill 0.3)
  Top 0.254: v12.38,58.42 11.43,59.37 C26.2
  Bottom 0.254: v12.38,58.42 12.38,56.52 BANDPASS3.2
N$32  (via drill 0.3)
  Top 0.254: R34.2 R35.1 C28.1 v11.43,58.42 | v20.48,57.31 20.48,57.47 20.16,57.79 19.37,57.79 IC4.12
  Bottom 0.254: v20.48,57.31 17.3,54.13 11.43,54.13 v11.43,58.42
N$33
  Top 0.254: IC5.7 26.5,47.67 R38.2 28.36,48.69 R37.2
N$34  (via drill 0.3)
  Top 0.254: R39.1 30.16,44.45 30.16,45.56 30.96,46.36 30.96,48.74 30.16,49.53 R38.1 30,49.53 28.89,50.64 v28.26,50.64 | v27.94,48.26 26.67,46.99 25.24,46.99 IC5.6
  Bottom 0.254: v28.26,50.64 28.26,49.53 GAIN4.2 28.1,49.53 28.1,48.42 v27.94,48.26
N$35
  Top 0.254: IC5.1 27.68,43.77 R39.2 R40.2
N$36  (via drill 0.3)
  Top 0.254: R41.2 16.05,43.77 17.78,43.77 | 17.78,43.77 18.1,43.77 | 18.1,43.77 IC5.14 19.37,43.82 19.37,44.29 IC5.13 | v17.78,42.23 18.73,41.27 R45.2 | v17.78,43.66 17.78,43.77 | 18.1,43.77 18.1,46.04 18.41,46.36 19.21,46.36 IC5.10
  Bottom 0.254: v17.78,43.66 v17.78,42.23
N$37  (via drill 0.3)
  Top 0.254: v16.35,44.61 15.24,44.61 R41.1 | v22.23,40.32 v19.68,40.32 | v28.89,40.8 30,41.91 R40.1 | v26.51,44.45 25.24,44.45 IC5.2
  Bottom 0.254: v16.35,44.61 19.68,44.61 v19.68,40.32 | 26.35,44.45 25.8,43.89 | 25.8,43.89 v22.23,40.32 | 26.35,44.45 26.35,49.53 GAIN4.1 | 25.8,43.89 v28.89,40.8 | 26.35,44.45 v26.51,44.45
N$38  (via drill 0.3)
  Top 0.254: v29.21,45.4 28.42,46.2 28.42,46.99 R37.1 | v22.38,51.28 C29.2
  Bottom 0.254: v29.21,45.4 29.21,50.64 28.1,51.75 24.61,51.75 24.61,44.77 24.29,44.45 22.38,44.45 v22.38,51.28
N$39  (via drill 0.3)
  Top 0.254: v12.38,45.72 11.43,46.67 C33.2
  Bottom 0.254: v12.38,45.72 12.38,43.82 BANDPASS4.2
N$40  (via drill 0.3)
  Top 0.254: R43.2 R44.1 C35.1 v11.43,45.72 | v20.48,45.09 19.37,45.09 IC5.12
  Bottom 0.254: v20.48,45.09 16.83,45.09 16.67,45.24 15.4,45.24 15.4,43.5 14.76,42.86 13.34,42.86 13.34,45.72 12.7,46.36 11.43,46.36 v11.43,45.72
N$41
  Top 0.254: IC6.7 26.5,34.97 R46.2 28.36,35.99 R47.2
N$42  (via drill 0.3)
  Top 0.254: R48.1 30,31.75 30,32.7 28.42,34.29 R47.1 | v28.1,35.4 28.1,34.45 28.26,34.29 R47.1 | R47.1 25.24,34.29 IC6.6
  Bottom 0.254: v28.1,35.4 28.1,36.83 GAIN5.2
N$43
  Top 0.254: IC6.1 27.68,31.07 R48.2 R49.2
N$44
  Top 0.254: R50.2 17.78,30.27 | 17.78,30.27 18.48,30.27 IC6.14 | R54.2 18.84,30.62 IC6.14 | IC6.13 19.37,31.59 19.37,31.12 IC6.14 | 17.78,30.27 17.78,33.02 18.41,33.66 19.21,33.66 IC6.10
N$45  (via drill 0.3)
  Top 0.254: v16.67,32.07 15.24,32.07 R50.1 | v26.35,38.58 v20.32,38.58 | v28.73,28.1 28.89,28.1 30,29.21 R49.1 | v26.51,31.75 25.24,31.75 IC6.2
  Bottom 0.254: v16.67,32.07 20.32,35.72 v20.32,38.58 | v26.35,38.58 26.35,36.83 GAIN5.1 26.51,36.83 v26.51,31.75 26.51,30.32 v28.73,28.1
N$46  (via drill 0.3)
  Top 0.254: v27.46,39.85 30,37.31 30,36.83 R46.1 | v22.38,37.78 21.59,37.78 C36.2
  Bottom 0.254: v27.46,39.85 22.86,39.85 22.86,38.26 v22.38,37.78
N$47  (via drill 0.3)
  Top 0.254: v12.38,33.02 11.43,33.97 C40.2
  Bottom 0.254: v12.38,33.02 12.38,31.12 BANDPASS5.2
N$48  (via drill 0.3)
  Top 0.254: R52.2 R53.1 10.48,31.97 | 10.48,31.97 C42.1 | v13.97,27.62 19.53,27.62 19.68,27.78 19.68,29.37 20.48,30.16 20.48,32.07 20.16,32.39 19.37,32.39 IC6.12 | 10.48,31.97 v10.48,31.12
  Bottom 0.254: v10.48,31.12 v13.97,27.62
N$49
  Top 0.254: IC7.7 26.5,22.27 R55.2 28.36,23.29 R56.2
N$50  (via drill 0.3)
  Top 0.254: R57.1 30,19.05 30,20 28.42,21.59 R56.1 | v28.1,22.7 28.1,21.75 28.26,21.59 R56.1 | R56.1 25.24,21.59 IC7.6
  Bottom 0.254: v28.1,22.7 28.1,24.13 GAIN6.2
N$51
  Top 0.254: IC7.1 27.68,18.37 28.15,18.84 | 28.15,18.84 R57.2 | R58.2 28.36,18.63 28.15,18.84
N$52  (via drill 0.3)
  Top 0.254: R59.2 17.3,17.56 | 17.3,17.56 18.48,17.56 IC7.14 | R63.2 18.84,17.92 IC7.14 | IC7.13 19.37,18.89 19.37,18.41 IC7.14 | v17.3,18.57 17.3,17.56 | v17.94,20.48 18.41,20.95 19.21,20.95 IC7.10
  Bottom 0.254: v17.3,18.57 17.3,19.84 v17.94,20.48
N$53  (via drill 0.3)
  Top 0.254: R58.1 30,16.51 30,17.46 29.21,18.26 29.21,19.84 29.05,20 26.99,20 v26.51,19.53 26.04,19.05 25.24,19.05 IC7.2 | v17.94,19.05 17.78,19.21 15.24,19.21 R59.1
  Bottom 0.254: v17.94,19.05 26.35,19.05 26.35,19.53 | 26.35,19.53 26.35,24.13 GAIN6.1 | 26.35,19.53 v26.51,19.53
N$54  (via drill 0.3)
  Top 0.254: v25.88,27.15 27.15,25.88 28.26,25.88 30,24.13 R55.1 | v22.23,25.88 21.11,24.77 C43.2
  Bottom 0.254: v25.88,27.15 22.23,27.15 v22.23,25.88
N$55  (via drill 0.3)
  Top 0.254: v12.38,20.32 11.43,21.27 C47.2
  Bottom 0.254: v12.38,20.32 12.38,18.41 BANDPASS6.2
N$56  (via drill 0.3)
  Top 0.254: R61.2 R62.1 10.48,19.27 | 10.48,19.27 C49.1 | v15.4,20.32 15.72,20.32 16.35,19.69 19.21,19.69 IC7.12 | 10.48,19.27 v10.48,18.41
  Bottom 0.254: v15.4,20.32 15.24,20.16 15.24,17.94 14.76,17.46 10.48,17.46 v10.48,18.41
N$57
  Top 0.254: IC8.7 26.5,9.57 R64.2 28.36,10.59 R65.2
N$58  (via drill 0.3)
  Top 0.254: R66.1 30,6.35 30,7.3 28.42,8.89 R65.1 | v28.1,10 28.1,9.05 28.26,8.89 R65.1 | R65.1 25.24,8.89 IC8.6
  Bottom 0.254: v28.1,10 28.1,11.43 GAIN7.2
N$59
  Top 0.254: R67.2 R66.2 27.68,5.67 IC8.1
N$60
  Top 0.254: R68.2 17.78,4.87 | 17.78,4.87 18.48,4.87 18.84,5.22 | 18.84,5.22 IC8.14 19.37,5.71 19.37,6.19 IC8.13 | R72.2 18.84,5.22 | 17.78,4.87 17.78,7.62 18.41,8.26 19.21,8.26 IC8.10
N$61  (via drill 0.3)
  Top 0.254: v16.83,8.26 15.24,6.67 R68.1 | v30,4.92 30,3.81 R67.1 | v26.51,6.35 25.24,6.35 IC8.2
  Bottom 0.254: v16.83,8.26 21.59,8.26 21.59,4.45 21.91,4.13 26.35,4.13 26.35,4.92 | 26.35,6.35 26.35,11.43 GAIN7.1 | 26.35,6.35 26.35,4.92 | 26.35,4.92 v30,4.92 | 26.35,6.35 v26.51,6.35
N$62  (via drill 0.3)
  Top 0.254: v28.26,13.18 30,11.43 R64.1 | v22.23,13.18 21.11,12.06 C50.2
  Bottom 0.254: v22.23,13.18 v28.26,13.18
N$63  (via drill 0.3)
  Top 0.254: v12.38,7.62 11.43,8.57 C54.2
  Bottom 0.254: v12.38,7.62 12.38,5.71 BANDPASS7.2
N$64  (via drill 0.3)
  Top 0.254: R70.2 R71.1 10.48,6.56 | 10.48,6.56 C56.1 | v20.48,6.67 20.16,6.98 19.37,6.98 IC8.12 | 10.48,6.56 v10.48,5.71
  Bottom 0.254: v20.48,6.67 16.67,6.67 16.67,5.87 15.08,4.29 10.48,4.29 v10.48,5.71
N$65  (via drill 0.3)
  Top 0.254: v27.15,97.16 25.24,97.16 IC1.5 25.08,97.16 24.29,97.16 23.97,97.47 23.97,98.74 25.56,100.33 25.56,100.97 C1.2
  Bottom 0.254: v27.15,97.16 R74.1
N$67  (via drill 0.3)
  Top 0.254: v26.99,8.26 25.24,8.26 IC8.5 25.08,8.26 24.29,8.26 23.97,8.57 23.97,9.84 25.56,11.43 25.56,12.06 C51.2
  Bottom 0.254: v26.99,8.26 R77.1
N$68  (via drill 0.3)
  Top 0.254: v26.99,20.95 25.24,20.95 IC7.5 | v24.45,25.88 25.56,24.77 C44.2
  Bottom 0.254: v26.99,20.95 27.3,20.95 | 27.3,20.95 R78.1 | v24.45,25.88 27.3,25.88 27.3,20.95
N$69  (via drill 0.3)
  Top 0.254: v27.15,33.66 25.24,33.66 IC6.5 | v24.77,36.51 24.77,36.67 25.56,37.47 C37.2
  Bottom 0.254: 27.3,33.66 R79.1 | v24.77,36.51 25.56,37.31 25.56,38.73 26.04,39.21 27.3,39.21 27.3,33.66 | 27.3,33.66 v27.15,33.66
N$70  (via drill 0.3)
  Top 0.254: v26.99,46.36 25.24,46.36 IC5.5 | v26.51,51.12 26.51,50.96 25.72,50.16 C30.2
  Bottom 0.254: v26.99,46.36 27.3,46.36 | 27.3,46.36 R80.1 | v26.51,51.12 27.3,50.32 27.3,46.36
N$71  (via drill 0.3)
  Top 0.254: v27.15,59.06 25.24,59.06 IC4.5 | v24.77,61.91 24.77,62.07 25.56,62.86 C23.2
  Bottom 0.254: 27.3,59.06 R76.1 | v24.77,61.91 25.56,62.71 25.56,62.86 25.88,63.18 27.3,63.18 27.3,59.06 | 27.3,59.06 v27.15,59.06
N$72  (via drill 0.3)
  Top 0.254: v26.99,71.75 25.24,71.75 IC3.5 | v25.72,76.68 25.72,75.56 C16.2
  Bottom 0.254: v26.99,71.75 27.3,71.75 | 27.3,71.75 R75.1 | v25.72,76.68 27.3,76.68 27.3,71.75
REF  (via drill 0.3)
  Top 0.254: R72.1 21.27,3.18 v21.59,3.49 | v21.59,15.87 R63.1 | v20.48,26.03 20.48,28.58 R54.1 | v20.64,42.39 20.64,41.27 R45.1 | REFERENCE.2 REFERENCE.1 | v21.59,92.08 R7.1 | v22.23,53.98 R36.1 | v22.23,68.26 20.64,66.67 R27.1 | v20.64,76.84 20.64,79.38 R18.1
  Bottom 0.254: v21.59,3.49 30.64,3.49 30.64,7.78 30.16,8.26 R77.2 30,8.26 30,15.87 | 30,15.87 v21.59,15.87 19.05,15.87 16.67,18.26 16.67,22.23 v20.48,26.03 20.96,26.51 20.96,42.07 v20.64,42.39 | 30,15.87 30,20.95 R78.2 30.16,20.95 30.16,33.66 | 30.16,45.4 30.16,46.36 R80.2 | 30.16,45.4 30.16,33.66 | 30.16,45.4 REFERENCE.1 | 30.16,92.08 30.16,97.16 R74.2 | 30.16,92.08 30.16,84.45 | 30.16,92.08 v21.59,92.08 | v22.23,53.98 27.15,53.98 27.15,55.4 30,58.26 30,59.06 | 30,68.26 v22.23,68.26 22.23,69.37 21.43,70.17 21.43,76.04 v20.64,76.84 | 30,68.26 30,71.75 R75.2 30.16,71.75 30.16,84.45 | 30,68.26 30,59.06 | 30,59.06 R76.2 30.16,59.06 31.75,57.47 31.75,57.15 REFERENCE.2 | 30.16,84.45 R73.2 | 30.16,33.66 R79.2
S$1  (via drill 0.3)
  other vias: 2.54,36.83
S$2  (via drill 0.3)
  other vias: 2.54,38.73
S$3  (via drill 0.3)
  other vias: 2.54,31.12
S$4  (via drill 0.3)
  other vias: 2.54,26.03
S$5  (via drill 0.3)
  other vias: 2.54,68.58
S$6  (via drill 0.3)
  other vias: 2.54,63.5
S$7  (via drill 0.3)
  other vias: 2.54,95.25
S$8  (via drill 0.3)
  other vias: 2.54,86.36
S$9  (via drill 0.3)
  other vias: 2.54,79.38
S$10  (via drill 0.3)
  other vias: 2.54,19.05
S$11  (via drill 0.3)
  other vias: 2.54,9.53
S$12  (via drill 0.3)
  other vias: 36.83,83.19
S$13  (via drill 0.3)
  other vias: 36.83,85.73
S$14  (via drill 0.3)
  other vias: 35.56,86.36
S$15  (via drill 0.3)
  other vias: 36.83,87
S$16  (via drill 0.3)
  other vias: 36.83,20.95
S$17  (via drill 0.3)
  other vias: 36.83,19.05
S$18  (via drill 0.3)
  other vias: 34.92,18.41
S$19  (via drill 0.3)
  other vias: 36.83,17.15
S$20  (via drill 0.3)
  other vias: 33.65,17.15
S$21  (via drill 0.3)
  other vias: 32.38,15.87
S$22  (via drill 0.3)
  other vias: 36.83,15.24
S$23  (via drill 0.3)
  other vias: 36.2,19.69
S$24  (via drill 0.3)
  other vias: 36.2,85.09
S$25  (via drill 0.3)
  other vias: 34.92,86.36
S$26  (via drill 0.3)
  other vias: 33.65,87.63
S$27  (via drill 0.3)
  other vias: 32.38,88.27
S$28  (via drill 0.3)
  other vias: 36.83,88.9
S$29  (via drill 0.3)
  other vias: 35.56,87.63
S$30  (via drill 0.3)
  other vias: 35.56,88.9
S$31  (via drill 0.3)
  other vias: 33.65,88.9
S$32  (via drill 0.3)
  other vias: 8.26,102.23
S$33  (via drill 0.3)
  other vias: 12.7,102.23
S$34  (via drill 0.3)
  other vias: 17.14,102.23
S$35  (via drill 0.3)
  other vias: 17.14,90.17
S$36  (via drill 0.3)
  other vias: 19.05,64.77
S$37  (via drill 0.3)
  other vias: 17.14,39.37
S$38  (via drill 0.3)
  other vias: 6.99,15.87
VCC  (via drill 0.3)
  Top 0.305: IC6.4 23.97,33.02 | 23.97,33.02 23.65,33.02 23.34,32.7 23.34,31.27 24.92,29.69 24.92,28.58 C38.1 25.08,28.58 25.08,26.99 26.67,25.4 26.67,24.13 25.4,22.86 24.13,22.86 23.97,22.7 23.97,20.32 | IC5.4 23.97,45.72 | 23.97,45.72 23.65,45.72 23.34,45.4 23.34,43.97 24.92,42.39 24.92,41.27 C31.1 25.08,41.27 26.99,39.37 26.99,37.15 25.72,35.88 24.45,35.88 23.97,35.4 23.97,33.02 | 23.57,83.74 23.65,83.82 IC2.4 | 23.57,83.74 23.34,83.5 23.34,82.07 24.92,80.49 24.92,79.38 C10.1 25.08,79.38 25.08,78.26 26.67,76.68 26.67,74.93 25.4,73.66 24.13,73.66 23.97,73.5 23.97,71.12 | 24.92,92.08 24.92,93.19 23.34,94.77 23.34,96.2 23.65,96.52 IC1.4 | 24.92,92.08 24.92,90.96 22.86,88.9 22.86,87.31 23.5,86.68 23.5,83.82 23.57,83.74 | 24.92,92.08 C2.1 | IC4.4 23.97,58.42 | 23.97,58.42 23.65,58.42 23.34,58.1 23.34,56.67 24.92,55.09 24.92,53.98 C24.1 25.08,53.98 27.15,51.91 27.15,50.01 26.35,49.21 25.08,49.21 23.97,48.1 23.97,45.72 | IC3.4 23.97,71.12 | 23.97,71.12 23.65,71.12 23.34,70.8 23.34,69.37 24.92,67.79 24.92,66.67 C17.1 25.08,66.67 26.67,65.09 26.67,62.23 25.72,61.28 24.45,61.28 23.97,60.8 23.97,58.42 | R16.1 9.53,86.68 12.86,90.01 12.86,90.17 | v13.34,96.52 C5.1 | v10.48,98.42 9.53,99.38 R10.1 9.53,99.22 8.41,99.22 7.94,98.74 7.94,80.96 11.99,76.91 | v11.43,92.71 11.43,90.33 C59.1 | 8.65,54.85 5.08,58.42 5.08,69.37 | 8.65,54.85 8.89,54.61 13.97,54.61 14.29,54.93 14.29,56.36 13.34,57.31 C25.1 | 5.08,69.37 5.08,70.48 PAD4.1 PAD3.1 | 5.08,69.37 9.53,73.82 | 9.53,73.82 10.48,72.87 10.48,71.44 10.79,71.12 12.07,71.12 13.02,70.17 13.34,70.17 C18.1 | 9.53,73.82 R25.1 9.53,74.45 11.99,76.91
  Top 0.305: 11.99,76.91 14.29,79.22 14.29,81.76 13.34,82.71 C11.1 | R70.1 9.53,10.48 12.86,13.81 12.86,13.97 | v14.76,7.62 14.61,7.62 13.65,6.67 13.34,6.67 C52.1 | C66.2 13.65,13.81 v15.56,11.91 17.46,11.91 18.41,10.95 22.86,10.95 | v14.29,16.51 14.29,18.26 13.34,19.21 C46.1 | 24.21,7.54 24.29,7.62 IC8.4 | 24.21,7.54 23.97,7.3 23.97,5.24 24.92,4.29 24.92,3.18 C53.1 | 24.92,15.87 24.92,16.99 23.34,18.57 23.34,20 23.65,20.32 23.97,20.32 | IC7.4 23.97,20.32 | 24.21,7.54 22.86,8.89 22.86,10.95 | 22.86,10.95 22.86,13.81 24.92,15.87 | 24.92,15.87 C45.1 | R61.1 9.53,24.77 14.21,29.45 | 14.21,29.45 14.29,29.53 14.29,30.96 13.34,31.91 C39.1 | 12.86,64.77 12.86,64.61 9.53,61.28 R34.1 9.53,61.12 10.48,60.17 v10.48,58.26 | R52.1 9.53,35.88 12.86,39.21 12.86,39.37 | v14.29,42.07 14.29,43.66 13.34,44.61 C32.1 | v13.81,40.64 13.81,39.37 C64.2 | v8.41,47.31 9.53,48.42 R43.1 | v14.29,29.37 14.21,29.45 | v8.57,54.77 8.65,54.85
  Top 0.356: C59.1 12.86,90.17 C60.2 | C65.1 12.86,13.97 C66.2 | C63.1 12.86,39.37 C64.2 | C61.1 12.86,64.77 C62.2
  Bottom 0.305: v13.34,96.52 12.54,97.31 11.43,97.31 | 11.43,97.31 10.48,97.31 v10.48,98.42 | 11.43,97.31 v11.43,92.71 | v14.76,7.62 15.56,8.41 v15.56,11.91 15.56,15.24 14.53,16.27 | 14.53,16.27 v14.29,16.51 | v14.29,42.07 13.81,41.59 13.81,40.8 | 13.81,40.8 11.59,43.02 11.59,44.13 v8.41,47.31 8.57,47.31 v8.57,54.77 8.57,56.36 v10.48,58.26 | 13.81,40.8 v13.81,40.64 15.72,38.73 15.72,30.8 v14.29,29.37 14.45,29.37 16.03,27.78 16.03,17.78 14.53,16.27

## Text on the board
Top: VCC | GND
